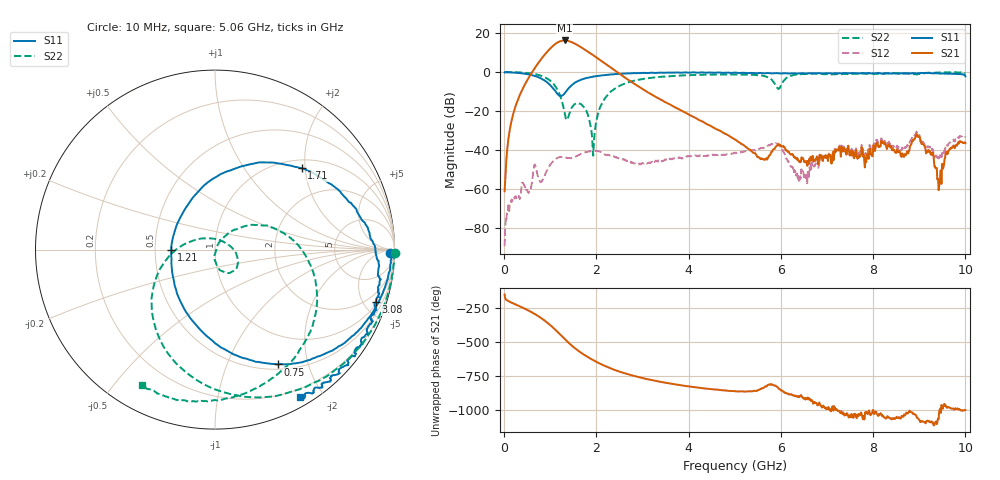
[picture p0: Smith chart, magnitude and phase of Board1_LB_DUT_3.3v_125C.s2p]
! Created Tue May 27 17:13:09 2025
# hz S ma R 50
! 2 Port Network Data from SP1.SP block
! freq  magS11  angS11  magS21  angS21  magS12  angS12  magS22  angS22
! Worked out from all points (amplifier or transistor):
!   1000 points, 10 MHz to 10 GHz, reference 50 ohm
!   highest |S21| = 16.2 dB at 1.31 GHz (marker M1)
!   |S21| within 3 dB of that: 1.048 GHz to 1.635 GHz (586.9 MHz wide, 43.7 % of centre)
!   unconditionally stable (mu >= 1): 15.78 MHz to 48.35 MHz; 51.14 MHz to end of sweep
!   at 1.67 GHz: K = 8.72, MAG = 15.0 dB, |S12| = -42.1 dB
!   at 5.01 GHz: K = 54.29, MAG = -17.0 dB, |S12| = -41.5 dB
!   at 10 GHz: K = 93.84, MAG = -24.1 dB, |S12| = -33.7 dB
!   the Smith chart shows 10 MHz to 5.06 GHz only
!   S11 on the Smith chart (normalised r, x): 10 MHz: 53, -32; 750 MHz: 0.56, -1.54; 1.21 GHz: 0.61, -0.00; 1.71 GHz: 1.19, +1.92; 3.08 GHz: 1.18, -6.10; 5.06 GHz: 0.10, -1.72
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1e7  0.9727 -1.0  0.0008618 -147.5  3.342e-05 0.5  1.004 -0.9
2.2e8  0.9636 -15.0  0.1036 141.9  0.0005918 80.0  0.9907 -19.7
7.5e8  0.7297 -61.3  1.761 49.7  0.001763 60.6  0.8372 -78.4
9e8  0.5793 -81.6  2.985 13.6  0.0025 111.8  0.713 -101.5
1.04e9  0.4074 -109.6  4.489 -26.0  0.004724 99.1  0.5397 -128.4
1.12e9  0.3117 -134.0  5.366 -51.5  0.005864 87.1  0.4131 -147.0
1.21e9  0.2443 -179.4  6.142 -82.0  0.006493 72.2  0.2529 -173.0
1.31e9  0.2823 125.8  6.47 -116.4  0.006464 59.8  0.09239 137.4
1.47e9  0.4611 76.8  5.817 -167.3  0.006228 56.1  0.1231 -13.2
1.68e9  0.6414 46.0  4.239 137.9  0.007982 48.9  0.1449 -63.0
1.71e9  0.6622 43.1  4.03 131.1  0.008185 46.6  0.1321 -68.9
1.93e9  0.7639 25.9  2.708 86.1  0.009401 26.0  0.007071 -13.9
2.12e9  0.8186 15.3  1.881 53.3  0.008548 5.4  0.1554 45.7
2.5e9  0.8939 -1.1  0.9038 0.9  0.006124 -5.4  0.4406 6.6
3.08e9  0.9419 -18.0  0.3187 -53.2  0.004589 6.6  0.684 -37.0
3.34e9  0.9568 -24.3  0.2117 -71.3  0.005168 8.7  0.7418 -52.3
5.01e9  0.9666 -59.2  0.01825 -144.7  0.008387 -10.4  0.8621 -116.4
5.06e9  0.9492 -60.1  0.01646 -146.4  0.008538 -9.4  0.8575 -118.3
6.67e9  0.93 -89.8  0.005933 148.6  0.004079 141.1  0.9065 -150.1
8.34e9  0.9132 -134.3  0.0141 21.3  0.01616 32.7  0.923 172.9
9.44e9  0.913 -166.2  0.001488 77.6  0.006771 63.4  0.9681 168.4
1e10  0.7747 176.5  0.01495 76.6  0.02065 67.8  0.9252 168.7
